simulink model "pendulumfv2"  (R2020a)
settings: Solver=ode45  StartTime=0.0  StopTime=10  RelTol=1e-3  EnableMultiTasking=on
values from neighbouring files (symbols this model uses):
  f = 0.3    [pendulumdemo.m]
  q10 = pi*theta0/180    (= 2.09439510239)    [pendulumdemo.m]
  q1L0 = q10    (= 2.09439510239)    [pendulumdemo.m]
  q20 = 0    [pendulumdemo.m]
  q2L0 = 0    [pendulumdemo.m]

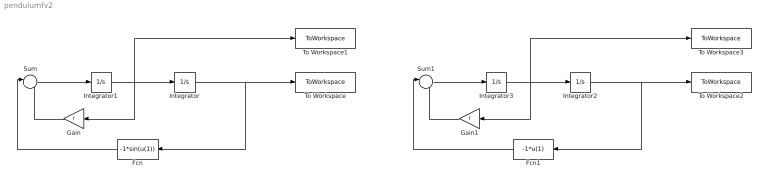
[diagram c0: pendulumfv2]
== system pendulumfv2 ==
  Fcn : Fcn  Expr=-1*sin(u(1))
  Fcn1 : Fcn  Expr=-1*u(1)
  Gain : Gain  Gain=f
  Gain1 : Gain  Gain=f
  Integrator : Integrator  InitialCondition=q10
  Integrator1 : Integrator  InitialCondition=q20
  Integrator2 : Integrator  InitialCondition=q1L0
  Integrator3 : Integrator  InitialCondition=q2L0
  Sum : Sum  Inputs=|+-
  Sum1 : Sum  Inputs=|+-
  To Workspace : ToWorkspace  VariableName=q1  SampleTime=-1
  To Workspace1 : ToWorkspace  VariableName=q2  SampleTime=-1
  To Workspace2 : ToWorkspace  VariableName=q1L  SampleTime=-1
  To Workspace3 : ToWorkspace  VariableName=q2L  SampleTime=-1
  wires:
  Integrator1/1 -> Gain/1, To Workspace1/1, Integrator/1
  Integrator/1 -> To Workspace/1, Fcn/1
  Fcn/1 -> Sum/1
  Sum/1 -> Integrator1/1
  Gain/1 -> Sum/2
  Integrator3/1 -> Gain1/1, To Workspace3/1, Integrator2/1
  Sum1/1 -> Integrator3/1
  Gain1/1 -> Sum1/2
  Fcn1/1 -> Sum1/1
  Integrator2/1 -> To Workspace2/1, Fcn1/1
